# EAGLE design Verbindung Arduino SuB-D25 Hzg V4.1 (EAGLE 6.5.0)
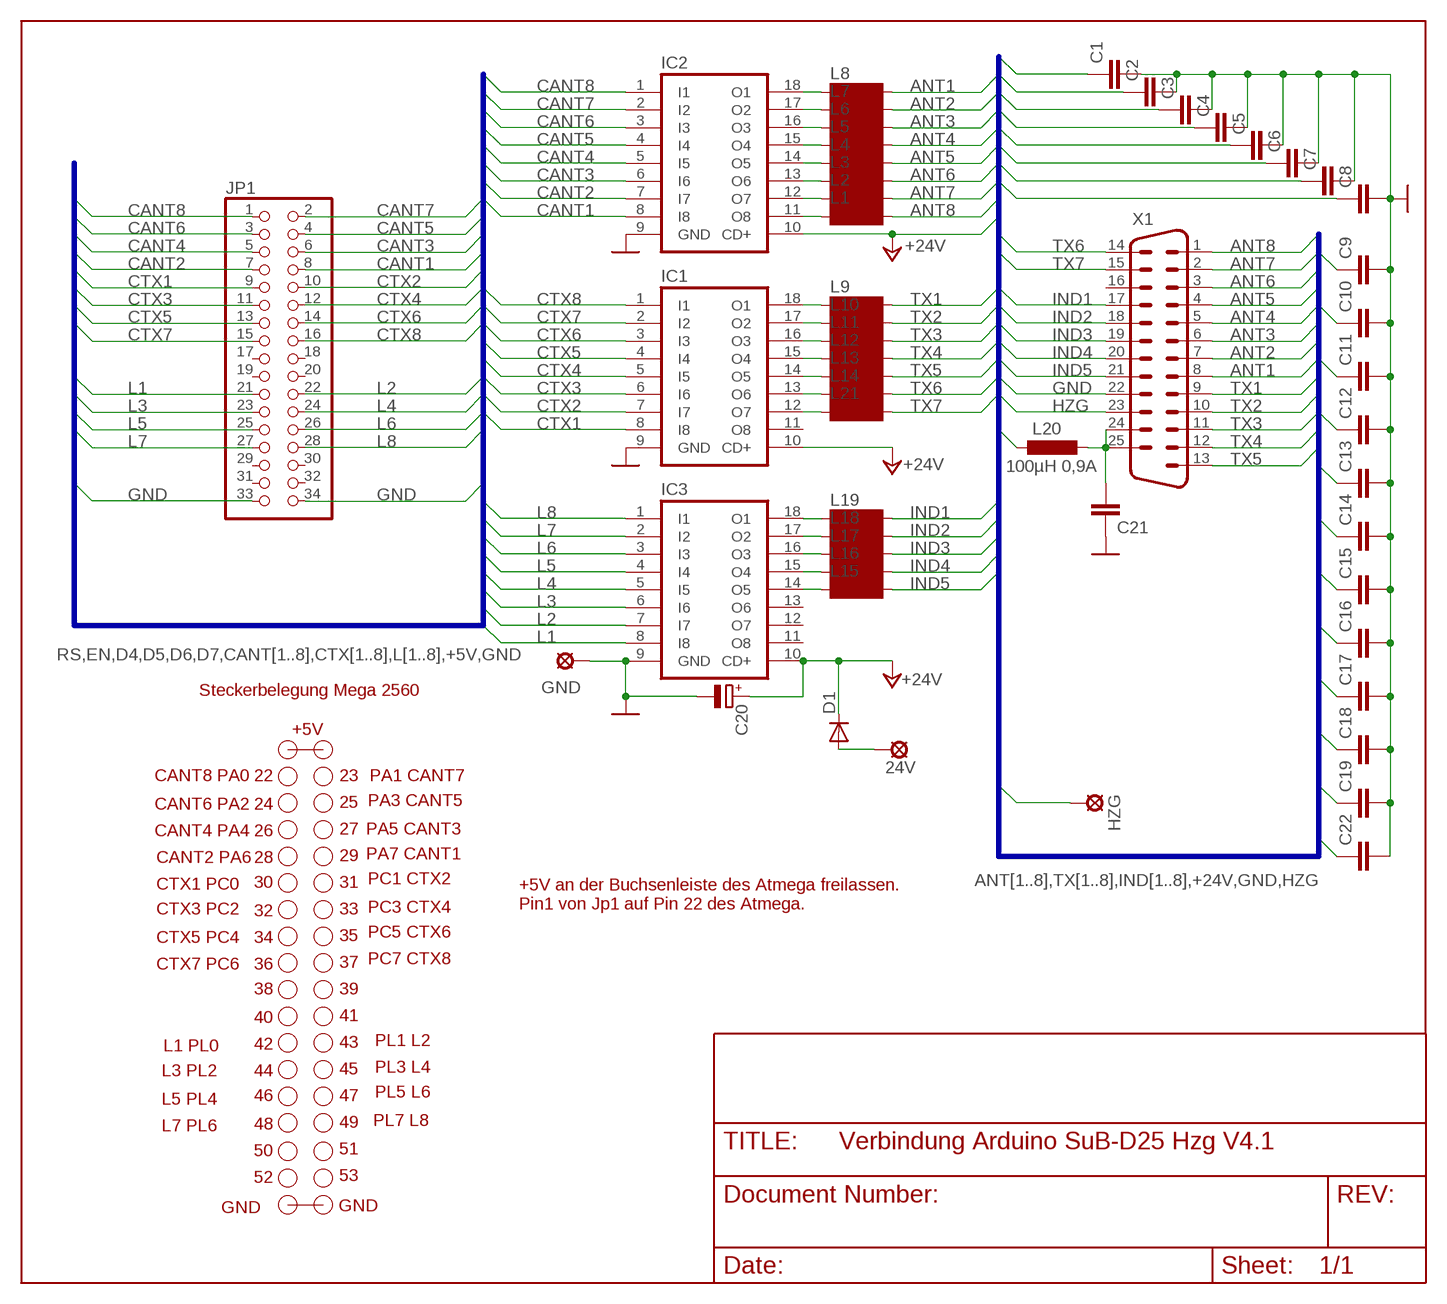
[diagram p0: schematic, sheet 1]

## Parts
24V  LSP13  [LSP13]
C1  C-EUC1206  [C1206]
C2  C-EUC1206  [C1206]
C3  C-EUC1206  [C1206]
C4  C-EUC1206  [C1206]
C5  C-EUC1206  [C1206]
C6  C-EUC1206  [C1206]
C7  C-EUC1206  [C1206]
C8  C-EUC1206  [C1206]
C9  C-EUC1206  [C1206]
C10  C-EUC1206  [C1206]
C11  C-EUC1206  [C1206]
C12  C-EUC1206  [C1206]
C13  C-EUC1206  [C1206]
C14  C-EUC1206  [C1206]
C15  C-EUC1206  [C1206]
C16  C-EUC1206  [C1206]
C17  C-EUC1206  [C1206]
C18  C-EUC1206  [C1206]
C19  C-EUC1206  [C1206]
C20  CPOL-EUSMCE  [SMC_E]
C21  C-EUC1206  [C1206]
C22  C-EUC1206  [C1206]
D1  DIODE-DO214BA  [DO214BA]
GND  LSP13  [LSP13]
HZG  LSP13  [LSP13]
IC1  ULN2803A  [DIL18]
IC2  ULN2803A  [DIL18]
IC3  ULN2803A  [DIL18]
JP1  PINHD-2X17  [2X17]
L1  SM-1206  [SM-1206]
L2  SM-1206  [SM-1206]
L3  SM-1206  [SM-1206]
L4  SM-1206  [SM-1206]
L5  SM-1206  [SM-1206]
L6  SM-1206  [SM-1206]
L7  SM-1206  [SM-1206]
L8  SM-1206  [SM-1206]
L9  SM-1206  [SM-1206]
L10  SM-1206  [SM-1206]
L11  SM-1206  [SM-1206]
L12  SM-1206  [SM-1206]
L13  SM-1206  [SM-1206]
L14  SM-1206  [SM-1206]
L15  SM-1206  [SM-1206]
L16  SM-1206  [SM-1206]
L17  SM-1206  [SM-1206]
L18  SM-1206  [SM-1206]
L19  SM-1206  [SM-1206]
L20  100µH 0,9A  L-EU  [242418FPS]
L21  SM-1206  [SM-1206]
X1  M25HP  [M25HP]

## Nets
+24V: C20.+ D1.C IC1.10(CD+) IC2.10(CD+) IC3.10(CD+) L20.1
ANT1: C8.1 L8.2 X1.8
ANT2: C7.1 L7.2 X1.7
ANT3: C6.1 L6.2 X1.6
ANT4: C5.1 L5.2 X1.5
ANT5: C4.1 L4.2 X1.4
ANT6: C3.1 L3.2 X1.3
ANT7: C2.1 L2.2 X1.2
ANT8: C1.1 L1.2 X1.1
CANT1: IC2.8(I8) JP1.8
CANT2: IC2.7(I7) JP1.7
CANT3: IC2.6(I6) JP1.6
CANT4: IC2.5(I5) JP1.5
CANT5: IC2.4(I4) JP1.4
CANT6: IC2.3(I3) JP1.3
CANT7: IC2.2(I2) JP1.2
CANT8: IC2.1(I1) JP1.1
CTX1: IC1.8(I8) JP1.9
CTX2: IC1.7(I7) JP1.10
CTX3: IC1.6(I6) JP1.11
CTX4: IC1.5(I5) JP1.12
CTX5: IC1.4(I4) JP1.13
CTX6: IC1.3(I3) JP1.14
CTX7: IC1.2(I2) JP1.15
CTX8: IC1.1(I1) JP1.16
GND: C1.2 C2.2 C3.2 C4.2 C5.2 C6.2 C7.2 C8.2 C9.2 C10.2 C11.2 C12.2 C13.2 C14.2 C15.2 C16.2 C17.2 C18.2 C19.2 C20.- C21.1 C22.2 GND.MP IC1.9(GND) IC2.9(GND) IC3.9(GND) JP1.33 JP1.34 X1.22
HZG: HZG.MP X1.23
IND1: C15.1 L19.2 X1.17
IND2: C16.1 L18.2 X1.18
IND3: C17.1 L17.2 X1.19
IND4: C18.1 L16.2 X1.20
IND5: C19.1 L15.2 X1.21
L1: IC3.8(I8) JP1.21
L2: IC3.7(I7) JP1.22
L3: IC3.6(I6) JP1.23
L4: IC3.5(I5) JP1.24
L5: IC3.4(I4) JP1.25
L6: IC3.3(I3) JP1.26
L7: IC3.2(I2) JP1.27
L8: IC3.1(I1) JP1.28
N$1: IC2.18(O1) L8.1
N$2: IC2.17(O2) L7.1
N$3: IC2.16(O3) L6.1
N$4: IC2.15(O4) L5.1
N$5: IC2.14(O5) L4.1
N$6: IC2.13(O6) L3.1
N$7: IC2.12(O7) L2.1
N$8: IC2.11(O8) L1.1
N$9: IC1.16(O3) L11.1
N$10: IC1.15(O4) L12.1
N$11: IC1.14(O5) L13.1
N$12: IC1.13(O6) L14.1
N$13: IC1.17(O2) L10.1
N$14: IC1.18(O1) L9.1
N$15: IC3.15(O4) L16.1
N$16: IC3.14(O5) L15.1
N$17: IC3.16(O3) L17.1
N$18: IC3.17(O2) L18.1
N$19: IC3.18(O1) L19.1
N$20: C21.2 L20.2 X1.24 X1.25
N$21: 24V.MP D1.A
N$22: IC1.12(O7) L21.1
TX1: C9.1 L9.2 X1.9
TX2: C10.1 L10.2 X1.10
TX3: C11.1 L11.2 X1.11
TX4: C12.1 L12.2 X1.12
TX5: C13.1 L13.2 X1.13
TX6: C14.1 L14.2 X1.14
TX7: C22.1 L21.2 X1.15
Unconnected: IC1.11(O8) IC3.11(O8) IC3.12(O7) IC3.13(O6) JP1.17 JP1.18 JP1.19 JP1.20 JP1.29 JP1.30 JP1.31 JP1.32 X1.16 X1.G1 X1.G2

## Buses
RS,EN,D4,D5,D6,D7,CANT[1..8],CTX[1..8],L[1..8],+5V,GND
ANT[1..8],TX[1..8],IND[1..8],+24V,GND,HZG

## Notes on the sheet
- Steckerbelegung Mega 2560
- +5V
- CANT8 PA0 | 22 | 23 | PA1 CANT7
- CANT6 PA2 | 24 | 25 | PA3 CANT5
- CANT4 PA4 | 26 | 27 | PA5 CANT3
- CANT2 PA6 | 28 | 29 | PA7 CANT1
- 30 | 31 | PC1 CTX2
- CTX1 PC0
- +5V an der Buchsenleiste des Atmega freilassen. 
  Pin1 von Jp1 auf Pin 22 des Atmega.
- CTX3 PC2 | 32 | 33 | PC3 CTX4
- 35 | PC5 CTX6
- CTX5 PC4 | 34
- 37 | PC7 CTX8
- CTX7 PC6 | 36
- 38 | 39
- 40 | 41
- 42 | 43 | PL1 L2
- L1 PL0
- L3 PL2 | 44 | 45 | PL3 L4
- 46 | 47 | PL5 L6
- L5 PL4
- 48 | 49 | PL7 L8
- L7 PL6
- 50 | 51
- 52 | 53
- GND | GND

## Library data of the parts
24V GND HZG = solpad:LSP13: SOLDER PAD
C1-C19 C21 C22 = rcl:C-EU: CAPACITOR, European symbol
C20 = rcl:CPOL-EU: POLARIZED CAPACITOR, European symbol
D1 = diode:DIODE-: DIODE
IC1-IC3 = uln-udn:ULN2803A: DRIVER ARRAY
JP1 = pinhead+:PINHD-2X17: PIN HEADER
L1-L19 L21 = inductor-neosid:SM-1206: INDUCTOR; OC_FARNELL: unknown; OC_NEWARK: unknown
L20 = rcl:L-EU: INDUCTOR, European symbol 100µH 242418FPS Reichelt
X1 = con-subd:M25HP: SUB-D; OC_FARNELL: unknown; OC_NEWARK: unknown

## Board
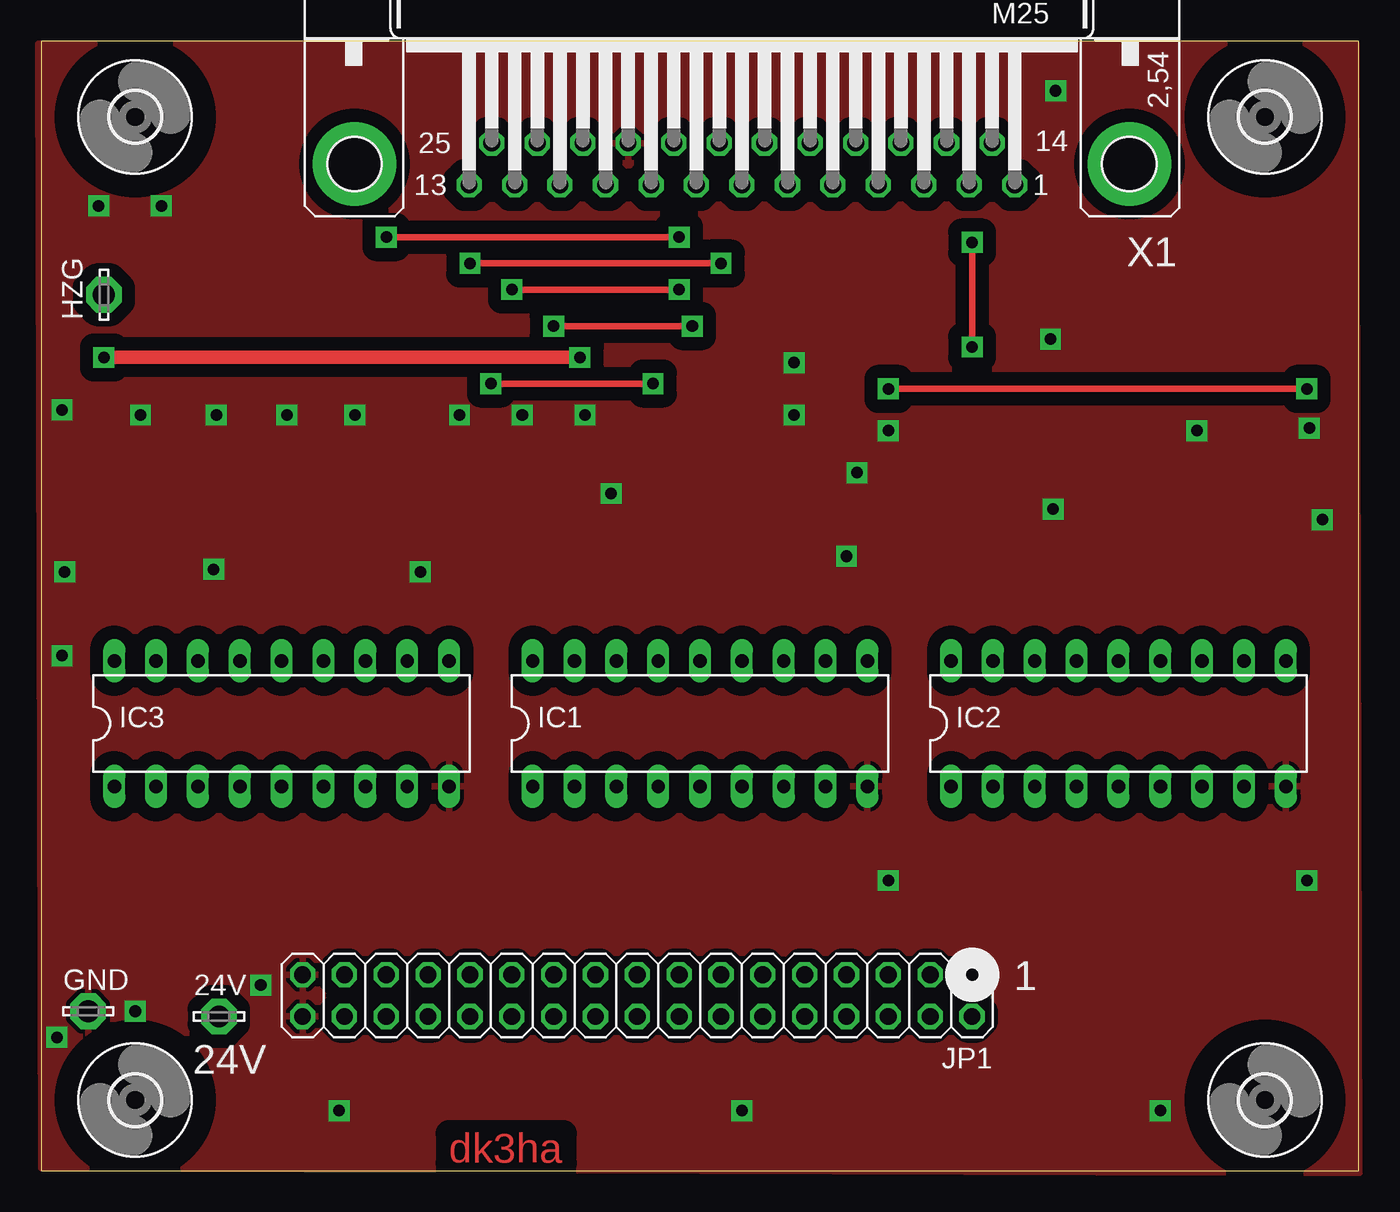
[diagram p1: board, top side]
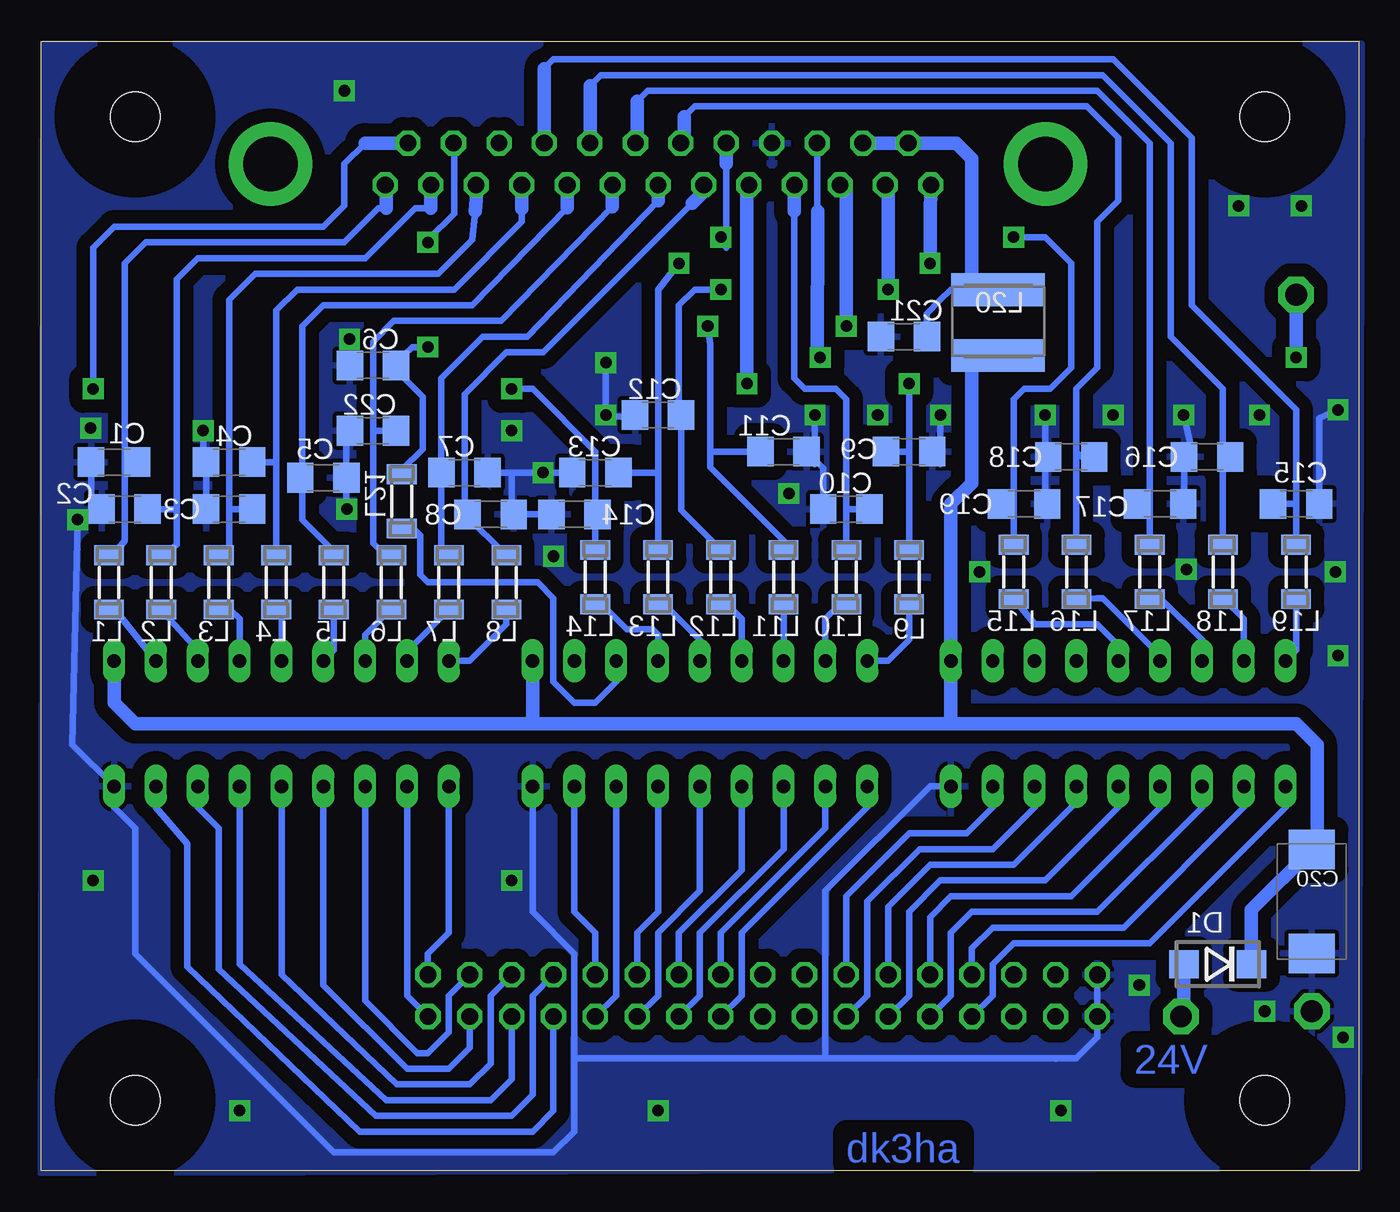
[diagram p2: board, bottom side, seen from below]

Size 79.99 x 68.57 mm. Coordinates in mm from the lower left corner, seen from the top.
Outline: 0,0 79.99,0 79.99,68.57 0,68.57 0,0
Copper layers (1*16): Top 0.035mm / dielectric 1.5mm / Bottom 0.035mm
Design rules "default *": minimum track width 10mil, minimum drill 24mil, track to track 8mil, track to pad 8mil, pad to pad 8mil, via to via 8mil, smd to smd 8mil, copper to edge 0mil, drill to drill 8mil, minimum pad ring 10mil, minimum via ring 8mil, stop-mask expansion 4mil, vias tented up to drill 0mil, thermal gap 10mil

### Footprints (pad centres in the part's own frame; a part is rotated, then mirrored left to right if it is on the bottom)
LSP13 = drill 1.321 pad 2.159 octagon: MP 0,0
C1206 = smd 1.6 x 1.8: 1 -1.4,0; 2 1.4,0
SMC_E = smd 2.4 x 2.8: + -3.15,0; - 3.15,0
DO214BA = smd 1.8 x 1.7: A 2.05,0; C -2.05,0
DIL18 = drill 0.813 long: 1 -10.16,-3.81; 2 -7.62,-3.81; 3 -5.08,-3.81; 4 -2.54,-3.81; 5 0,-3.81; 6 2.54,-3.81; 7 5.08,-3.81; 8 7.62,-3.81; 9 10.16,-3.81; 10 10.16,3.81; 11 7.62,3.81; 12 5.08,3.81; 13 2.54,3.81; 14 0,3.81; 15 -2.54,3.81; 16 -5.08,3.81; 17 -7.62,3.81; 18 -10.16,3.81
2X17 = drill 1.016 octagon: 1 -20.32,-1.27; 2 -20.32,1.27; 3 -17.78,-1.27; 4 -17.78,1.27; 5 -15.24,-1.27; 6 -15.24,1.27; 7 -12.7,-1.27; 8 -12.7,1.27; 9 -10.16,-1.27; 10 -10.16,1.27; 11 -7.62,-1.27; 12 -7.62,1.27; 13 -5.08,-1.27; 14 -5.08,1.27; 15 -2.54,-1.27; 16 -2.54,1.27; 17 0,-1.27; 18 0,1.27; 19 2.54,-1.27; 20 2.54,1.27; 21 5.08,-1.27; 22 5.08,1.27; 23 7.62,-1.27; 24 7.62,1.27; 25 10.16,-1.27; 26 10.16,1.27; 27 12.7,-1.27; 28 12.7,1.27; 29 15.24,-1.27; 30 15.24,1.27; 31 17.78,-1.27; 32 17.78,1.27; 33 20.32,-1.27; 34 20.32,1.27
SM-1206 = smd 1.2 x 1.8: 1 -1.65,0; 2 1.65,0
242418FPS = smd 2 x 5.7: 1 -2.1,0; 2 1.9,0
3,0 = hole 3: 0,0
M25HP = drill 1.016 octagon: 1 -16.561,1.27; 2 -13.792,1.27; 3 -11.049,1.27; 4 -8.28,1.27; 5 -5.512,1.27; 6 -2.769,1.27; 7 0,1.27; 8 2.769,1.27; 9 5.512,1.27; 10 8.28,1.27; 11 11.049,1.27; 12 13.792,1.27; 13 16.561,1.27; 14 -15.189,-1.27; 15 -12.421,-1.27; 16 -9.652,-1.27; 17 -6.909,-1.27; 18 -4.14,-1.27; 19 -1.372,-1.27; 20 1.372,-1.27; 21 4.14,-1.27; 22 6.909,-1.27; 23 9.652,-1.27; 24 12.421,-1.27; 25 15.189,-1.27 | drill 3.302 pad 5.08: G1 -23.52,0; G2 23.52,0

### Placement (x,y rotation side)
24V  10.79,9.36 0 top
C1  75.56,43.02 180 bottom
C2  74.92,40.16 180 bottom
C3  68.57,40.16 180 bottom
C4  68.57,43.02 180 bottom
C5  62.86,42.06 0 bottom
C6  59.84,44.92 180 bottom
C7  54.29,42.38 0 bottom
C8  52.7,39.84 0 bottom
C9  27.3,43.65 0 bottom
C10  31.11,40.16 180 bottom
C11  34.92,43.65 0 bottom
C12  42.54,45.87 180 bottom
C13  46.35,42.38 180 bottom
C14  47.62,39.84 180 bottom
C15  3.81,40.48 0 bottom
C16  9.2,43.33 180 bottom
C17  12.06,40.48 0 bottom
C18  17.46,43.33 180 bottom
C19  20.32,40.48 0 bottom
C20  2.85,16.34 270 bottom
C21  27.62,50.63 0 bottom
C22  59.84,48.89 180 bottom
D1  8.57,12.54 180 bottom
GND  2.85,9.68 0 top
HZG  3.81,53.17 90 top
IC1  40,27.14 0 top
IC2  65.4,27.14 0 top
IC3  14.6,27.14 0 top
JP1  36.19,10.63 180 top
L1  75.88,35.71 90 bottom
L2  72.7,35.71 90 bottom
L3  69.21,35.71 90 bottom
L4  65.72,35.71 90 bottom
L5  62.23,35.71 90 bottom
L6  58.73,35.71 90 bottom
L7  55.24,35.71 90 bottom
L8  51.75,35.71 90 bottom
L9  27.3,36.03 90 bottom
L10  31.11,36.03 90 bottom
L11  34.92,36.03 90 bottom
L12  38.73,36.03 90 bottom
L13  42.54,36.03 90 bottom
L14  46.35,36.03 90 bottom
L15  20.95,36.35 90 bottom
L16  17.14,36.35 90 bottom
L17  12.7,36.35 90 bottom
L18  8.25,36.35 90 bottom
L19  3.81,36.35 90 bottom
L20  21.9,51.59 90 bottom
L21  58.1,40.63 90 bottom
U$1  [3,0]  5.71,63.97 0 top
U$2  [3,0]  74.29,4.28 0 top
U$3  [3,0]  5.71,4.28 0 top
U$4  [3,0]  74.29,63.97 0 top
X1  42.54,61.11 180 top

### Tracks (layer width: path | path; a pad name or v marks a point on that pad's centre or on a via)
+24V
  Bottom 0.813: 24.76,27.14 IC3.10 24.76,40.48 23.49,41.74 23.49,48.73 22.73,49.49 L20.1 | 24.76,27.14 50.16,27.14 | 50.16,27.14 74.29,27.14 75.56,28.41 IC2.10 | IC1.10 50.16,27.14 | 24.76,27.14 3.81,27.14 2.53,25.87 2.53,20.45 C20.+ 6.52,15.83 D1.C
ANT1
  Bottom 0.406: 54.29,39.84 54.29,47.14 51.75,49.68 49.52,49.68 40.48,58.73 | 54.29,39.84 L8.2 | C8.1 54.29,39.84
  Bottom 0.813: 40.48,58.73 39.84,59.37 39.84,59.77 X1.8
ANT2
  Bottom 0.406: 42.54,58.89 50.48,50.63 53.18,50.63 55.72,48.09 55.72,42.38 | 55.72,42.38 55.72,37.94 55.3,37.36 L7.2 | C7.1 55.72,42.38
  Bottom 0.813: X1.7 42.54,58.89
ANT3
  Bottom 0.406: 45.31,58.5 52.06,51.59 58.57,51.59 59.84,50.32 59.84,44.92 | 59.84,44.92 59.84,38.09 59.11,37.36 L6.2 | C6.1 59.84,44.92
  Bottom 0.813: X1.6 45.31,58.5
ANT4
  Bottom 0.406: 48.05,58.46 53.81,52.54 62.86,52.54 64.13,51.27 64.13,42.06 | 64.13,42.06 64.13,39.52 62.23,37.62 L5.2 | C5.1 64.13,42.06
  Bottom 0.813: X1.5 48.05,58.46
ANT5
  Bottom 0.406: 50.82,58.39 50.82,57.59 54.92,53.49 64.45,53.49 65.72,52.22 65.72,43.02 | 65.72,43.02 L4.2 | C4.1 65.72,43.02
  Bottom 0.813: X1.4 50.82,58.39
ANT6
  Bottom 0.406: 53.65,58.26 53.81,56.51 55.88,54.45 66.99,54.45 68.57,52.86 68.57,40.16 | 68.57,40.16 68.57,36.98 68.64,37.3 L3.2 | C3.1 68.57,40.16
  Bottom 0.813: X1.3 53.59,58.95 53.65,58.26
ANT7
  Bottom 0.406: 56.33,58.43 57.29,58.43 60.32,55.4 70.48,55.4 71.75,54.13 71.75,40.16 | 71.75,40.16 71.75,38 L2.2 | C2.1 71.75,40.16
  Bottom 0.813: X1.2 56.33,58.43
ANT8
  Bottom 0.406: L1.2 75.62,37.36 74.92,38.25 74.92,43.02 | 74.92,43.02 74.92,55.08 73.65,56.35 62.07,56.35 61.59,56.35 59.53,58.41 59.05,58.41 | 59.05,60.11 X1.1 | C1.1 74.92,43.02
  Bottom 0.813: 59.05,58.41 59.05,60.11
CANT1
  Bottom 0.406: IC2.8 73.02,22.06 71.11,19.84 71.11,12.38 60.64,2.38 50.16,2.38 48.89,3.65 JP1.8
CANT2
  Bottom 0.406: IC2.7 70.48,22.06 69.21,20.79 69.21,12.22 59.69,3.33 51.43,3.33 50.16,4.6 50.16,10.63 JP1.7
CANT3
  Bottom 0.406: IC2.6 67.94,12.54 59.05,4.28 52.7,4.28 51.43,5.55 JP1.6
CANT4
  Bottom 0.406: IC2.5 65.4,11.9 58.41,5.23 53.97,5.23 52.7,6.5 52.7,10.63 JP1.5
CANT5
  Bottom 0.406: IC2.4 62.86,11.27 57.78,6.19 55.24,6.19 53.97,7.46 JP1.4
CANT6
  Bottom 0.406: IC2.3 60.32,10.31 57.15,7.14 56.51,7.14 55.24,8.41 55.24,10.63 JP1.3
CANT7
  Bottom 0.406: IC2.2 57.78,10.63 JP1.2
CANT8
  Bottom 0.406: IC2.1 55.24,14.44 56.51,13.17 JP1.1
CTX1
  Bottom 0.406: IC1.8 47.62,15.71 46.35,14.44 JP1.9
CTX2
  Bottom 0.406: IC1.7 45.08,10.63 JP1.10
CTX3
  Bottom 0.406: IC1.6 42.54,15.71 43.81,14.44 JP1.11
CTX4
  Bottom 0.406: IC1.5 40,16.98 42.54,14.44 42.54,10.63 JP1.12
CTX5
  Bottom 0.406: IC1.4 37.46,18.25 41.27,14.44 JP1.13
CTX6
  Bottom 0.406: IC1.3 34.92,19.52 40,14.44 40,10.63 JP1.14
CTX7
  Bottom 0.406: IC1.2 32.38,20.79 38.73,14.44 JP1.15
CTX8
  Bottom 0.406: IC1.1 29.84,22.06 37.46,14.44 37.46,10.63 JP1.16
GND  (via drill 0.7 pad 1.27)
  Bottom 0.406: 18.41,6.82 17.14,6.82 15.87,8.09 JP1.34 JP1.33 | 18.41,6.82 32.38,6.82 | 32.38,6.82 32.38,16.98 26.03,23.33 IC3.9 | IC1.9 50.16,15.71 47.62,13.17 47.62,6.82 | 47.62,6.82 32.38,6.82 | 47.62,6.82 47.62,2.38 48.89,1.1 62.23,1.1 74.29,13.17 74.29,20.79 75.56,22.06 IC2.9 78.1,25.87 v77.78,39.52 76.83,39.84 76.51,40.16 | C6.2 61.27,44.92 61.27,44.6 61.46,44.6 C5.2 | 61.4,42.12 C5.2 | C3.2 C4.2 70.16,43.2 v70.16,44.92 | C1.2 76.96,40.6 76.51,40.16 | 76.51,40.16 C2.2 | 61.59,41.93 C5.2 | C14.2 C8.2 51.43,39.97 51.43,42.38 C7.2 v49.52,42.38 C13.2 | C12.2 43.94,45.69 v45.72,45.87 v45.72,49.05 | v45.72,49.05 45.72,49.37 46.03,49.05 v45.72,49.05 | C10.2 32.51,42.64 C11.2 33.02,42.88 v33.02,45.87 | v25.39,45.87 25.39,42.88 C9.2 | v10.63,45.87 10.16,43.78 C16.2 10.6,40.21 C17.2 | v19.05,45.87 19.05,43.65 | 19.05,43.65 19.05,40.29 C19.2 | C18.2 18.86,43.46 19.05,43.65 | C15.2 2.4,45.69 v1.27,46.19 | 18.39,6.79 18.41,6.82 | v61.43,40.16 61.46,40.16 C5.2
  other vias: 29.2,45.87 34.6,41.11 6.03,45.87 14.92,45.87 76.83,17.61 67.94,3.65 42.54,3.65 0.95,8.09 51.43,17.61 61.59,65.56 13.33,11.27 61.27,50.48 3.49,58.57 7.3,58.57 5.71,9.68 18.09,3.65 1.27,31.27 51.43,44.92 48.89,37.3 23.01,36.35 1.42,36.35 10.47,36.51 76.99,45.08
  pour Bottom (isolate 0.813): -0.16,68.42 79.85,68.42 80,-0.16 -0.01,0.15
  pour Top (isolate 0.813): -0.16,68.42 79.85,68.42 80,-0.16 -0.01,0.15
HZG  (via drill 0.7 pad 1.27)
  Top 0.813: v32.7,49.37 v3.81,49.37
  Bottom 0.406: X1.23 32.89,58.38 32.86,58.26 | 32.89,49.24 v32.7,49.37
  Bottom 0.813: 32.86,58.26 32.89,49.24 | v3.81,49.37 HZG.MP
IND1
  Bottom 0.406: 49.45,66.9 48.89,67.46 14.92,67.46 10.16,62.7 10.16,52.54 3.81,46.19 3.81,40.48 | L19.2 3.81,40.48 | C15.1 3.81,40.48
  Bottom 0.813: X1.17 49.45,66.9
IND2
  Bottom 0.406: L18.2 8.25,43.65 | 8.25,43.65 8.25,47.46 11.43,50.63 11.43,62.38 15.55,66.51 46.03,66.51 46.67,65.88 | 46.67,62.71 X1.18 | C16.1 7.93,43.33 8.25,43.65
  Bottom 0.813: 46.67,65.88 46.67,62.71
IND3
  Bottom 0.406: L17.2 12.7,39.84 | 12.7,39.84 12.7,62.38 15.87,65.56 43.17,65.56 43.81,64.92 | 43.81,62.8 X1.19 | C17.1 13.01,40.16 12.7,39.84
  Bottom 0.813: 43.81,64.92 43.81,62.8
IND4
  Bottom 0.406: L16.2 17.14,43.65 | 17.14,43.65 17.14,47.46 15.87,48.73 15.87,57.62 14.6,58.89 14.6,62.7 16.5,64.61 40.32,64.61 40.95,63.97 | 40.95,62.92 X1.20 | C18.1 16.82,43.33 17.14,43.65
  Bottom 0.813: 40.95,63.97 40.95,62.92
IND5  (via drill 0.7 pad 1.27)
  Top 0.406: v38.73,56.67 v20.95,56.67
  Bottom 0.406: 38.4,61.12 38.41,61.11 38.4,56.02 v38.73,56.67 | v20.95,56.67 19.05,56.67 17.46,55.08 17.46,48.73 18.73,47.46 20.32,47.46 20.95,46.83 20.95,39.84 | 20.95,39.84 L15.2 | C19.1 21.27,40.16 20.95,39.84
  Bottom 0.813: X1.21 38.4,61.12
L1
  Bottom 0.406: IC3.8 22.22,22.06 23.81,20.47 27.3,20.47 31.11,16.66 JP1.21
L2
  Bottom 0.406: IC3.7 19.68,22.06 22.22,19.52 26.66,19.52 29.84,16.34 29.84,10.63 JP1.22
L3
  Bottom 0.406: IC3.6 17.14,22.38 20.95,18.57 26.03,18.57 28.57,16.03 JP1.23
L4
  Bottom 0.406: JP1.24 27.3,10.63 27.3,15.71 25.39,17.61 19.05,17.61 14.6,22.06 IC3.5
L5
  Bottom 0.406: JP1.25 26.03,15.39 24.76,16.66 17.46,16.66 12.06,22.06 IC3.4
L6
  Bottom 0.406: JP1.26 24.76,10.63 24.76,14.44 23.49,15.71 15.87,15.71 9.52,22.06 IC3.3
L7
  Bottom 0.406: JP1.27 23.49,13.49 22.22,14.76 14.28,14.76 6.98,22.06 IC3.2
L8
  Bottom 0.406: JP1.28 22.22,10.63 22.22,12.54 20.95,13.8 12.7,13.8 4.44,22.06 IC3.1
N$1
  Bottom 0.406: L8.1 51.75,33.17 53.97,30.95 IC2.18
N$2
  Bottom 0.406: IC2.17 57.78,31.52 L7.1
N$3
  Bottom 0.406: L6.1 59.05,33.81 60.32,32.54 IC2.16
N$4
  Bottom 0.406: L5.1 62.23,31.59 IC2.15
N$5
  Bottom 0.406: L4.1 65.72,33.81 65.4,33.49 IC2.14
N$6
  Bottom 0.406: L3.1 68.51,34.06 67.94,33.49 IC2.13
N$7
  Bottom 0.406: L2.1 70.48,31.59 IC2.12
N$8
  Bottom 0.406: L1.1 75.56,34.12 IC2.11
N$9
  Bottom 0.406: L11.1 IC1.16
N$10
  Bottom 0.406: L12.1 38.35,34.38 37.46,33.49 IC1.15
N$11
  Bottom 0.406: L13.1 42.16,34.38 40,32.22 IC1.14
N$12
  Bottom 0.406: L14.1 45.97,34.38 44.45,32.85 42.86,32.85 42.54,32.54 IC1.13
N$13
  Bottom 0.406: L10.1 31.49,34.38 32.38,33.49 IC1.17
N$14
  Bottom 0.406: IC1.18 28.57,30.95 27.3,32.22 L9.1
N$15
  Bottom 0.406: L16.1 17.08,34.7 15.87,34.76 15.55,34.76 12.06,31.27 IC3.15
N$16
  Bottom 0.406: L15.1 20.95,34.76 19.68,33.17 15.87,33.17 14.6,31.9 IC3.14
N$17
  Bottom 0.406: L17.1 12,34.7 9.52,32.22 IC3.16
N$18
  Bottom 0.406: L18.1 8.19,34.7 6.98,33.49 IC3.17
N$19
  Bottom 0.406: L19.1 3.81,31.59 IC3.18
N$20
  Bottom 0.406: C21.2 26.22,52.03 25.39,52.86 24.77,53.49 L20.2
  Bottom 0.813: L20.2 22.54,53.17 23.49,54.13 23.49,61.43 24.44,62.38 X1.25 X1.24
N$21
  Bottom 0.813: D1.A 10.62,9.53 24V.MP
N$22
  Bottom 0.406: IC1.12 45.08,29.68 46.35,28.41 47.62,28.41 48.89,29.68 48.89,34.76 49.84,35.71 56.51,35.71 56.99,36.19 56.99,38.57 57.78,39.36 57.78,39.14 L21.1
TX1  (via drill 0.7 pad 1.27)
  Top 0.406: v27.3,47.78 v37.14,47.78
  Bottom 0.406: L9.2 27.3,43.65 | 27.3,43.65 v27.3,47.78 | 37.14,60.05 X1.9 | C9.1 27.3,43.65
  Bottom 0.813: v37.14,47.78 37.14,60.05
TX2
  Bottom 0.406: L10.2 31.11,40.16 | 31.11,40.16 31.11,46.83 31.74,47.46 33.65,47.46 34.29,48.09 34.29,58.26 | 34.29,60.13 X1.10 | C10.1 31.11,40.16
  Bottom 0.813: 34.29,58.26 34.29,60.13
TX3  (via drill 0.7 pad 1.27)
  Top 0.406: v39.52,51.27 v31.11,51.27
  Bottom 0.406: 31.11,59.78 X1.11 | L11.2 34.92,38.25 39.37,42.7 39.37,43.65 | 39.37,43.65 39.37,50.16 v39.52,51.27 | C11.1 39.37,43.65
  Bottom 0.813: v31.11,51.27 31.11,59.78
TX4  (via drill 0.7 pad 1.27)
  Top 0.406: v38.73,53.49 v28.57,53.49
  Bottom 0.406: 28.57,59.98 X1.12 | v38.73,53.49 40.32,53.49 41.27,52.54 41.27,46 C12.1 41.14,40.09 L12.2
  Bottom 0.813: v28.57,53.49 28.57,59.98
TX5  (via drill 0.7 pad 1.27)
  Top 0.406: v41.27,55.08 v26.03,55.08
  Bottom 0.406: L13.2 42.54,42.38 | 42.54,42.38 42.54,53.49 v41.27,55.08 | 25.98,60.11 26.03,60.11 X1.13 | C13.1 42.54,42.38
  Bottom 0.813: v26.03,55.08 26.03,57.62 25.98,60.11
TX6  (via drill 0.7 pad 1.27)
  Top 0.406: v51.43,47.46 v76.83,47.46
  Bottom 0.406: L14.2 46.35,39.84 | 46.35,39.84 46.35,43.65 50.16,47.46 v51.43,47.46 | v76.83,47.46 76.83,56.03 75.56,57.3 62.86,57.3 61.59,58.57 61.59,61.11 60.32,62.38 | C14.1 46.35,39.84
  Bottom 0.813: 60.32,62.38 X1.14
TX7  (via drill 0.7 pad 1.27)
  Top 0.406: v56.51,50 v56.51,56.35
  Bottom 0.406: L21.2 58.1,42.54 56.83,43.81 56.83,46.98 57.94,48.09 57.94,48.73 | 57.94,48.73 57.94,49.52 57.46,50 v56.51,50 | v56.51,56.35 56.51,56.51 54.92,58.1 54.92,62.34 X1.15 | C22.1 58.1,48.89 57.94,48.73

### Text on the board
Top: dk3ha
Bottom: 24V | dk3ha
tPlace: 1 | 24V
